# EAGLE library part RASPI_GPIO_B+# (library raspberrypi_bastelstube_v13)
2x20 header connector, all pins connected
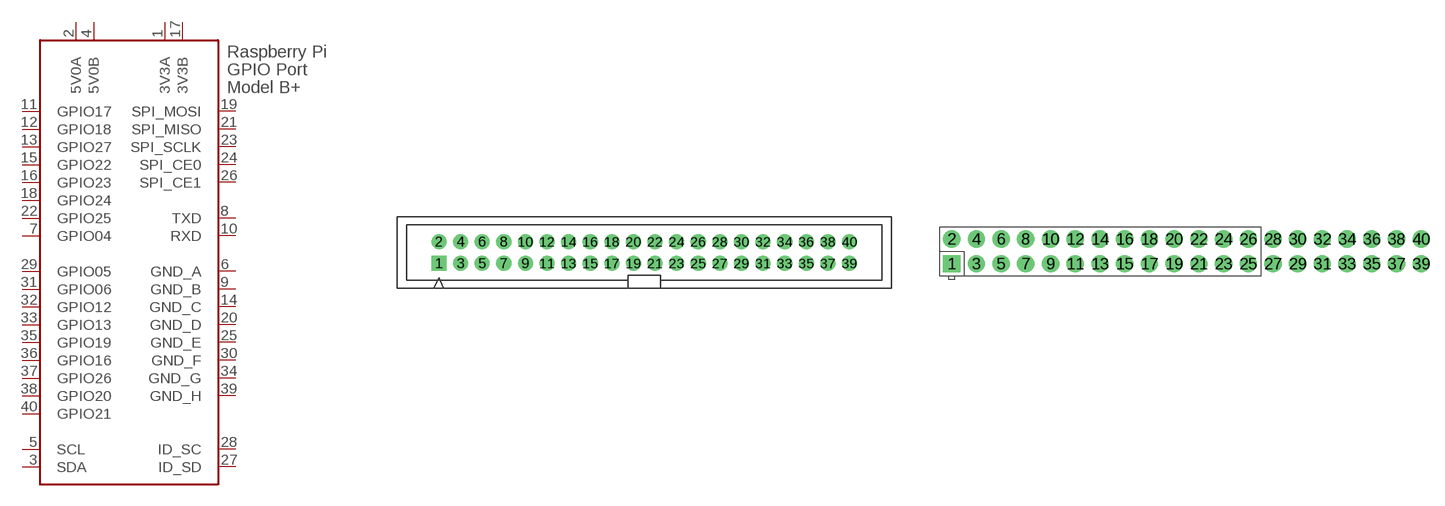
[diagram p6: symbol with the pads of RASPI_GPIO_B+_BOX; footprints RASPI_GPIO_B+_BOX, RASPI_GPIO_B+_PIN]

Designator prefix X

## RASPI_GPIO_B+#_BOX  [RASPI_GPIO_B+_BOX]
1  3V3A  pwr
2  5V0A  pwr
3  SDA
4  5V0B  pwr
5  SCL
6  GND_A  pwr
7  GPIO04
8  TXD
9  GND_B  pwr
10  RXD
11  GPIO17
12  GPIO18
13  GPIO27
14  GND_C  pwr
15  GPIO22
16  GPIO23
17  3V3B  pwr
18  GPIO24
19  SPI_MOSI
20  GND_D  pwr
21  SPI_MISO
22  GPIO25
23  SPI_SCLK
24  SPI_CE0
25  GND_E  pwr
26  SPI_CE1
27  ID_SD  nc
28  ID_SC  nc
29  GPIO05  nc
30  GND_F  pwr
31  GPIO06  nc
32  GPIO12  nc
33  GPIO13  nc
34  GND_G  pwr
35  GPIO19  nc
36  GPIO16  nc
37  GPIO26  nc
38  GPIO20  nc
39  GND_H  pwr
40  GPIO21  nc

## RASPI_GPIO_B+#_PIN  [RASPI_GPIO_B+_PIN]
Pads as for RASPI_GPIO_B+_BOX

## Footprint RASPI_GPIO_B+_BOX (pad centres in mm)
40-pin box header for Raspberry Pi GPIO model B+ for use with flat ribbon cables
drill 1 pad 1.778 square: 1 -24.13,-1.27
drill 1 pad 1.778: 2 -24.13,1.27; 3 -21.59,-1.27; 4 -21.59,1.27; 5 -19.05,-1.27; 6 -19.05,1.27; 7 -16.51,-1.27; 8 -16.51,1.27; 9 -13.97,-1.27; 10 -13.97,1.27; 11 -11.43,-1.27; 12 -11.43,1.27; 13 -8.89,-1.27; 14 -8.89,1.27; 15 -6.35,-1.27; 16 -6.35,1.27; 17 -3.81,-1.27; 18 -3.81,1.27; 19 -1.27,-1.27; 20 -1.27,1.27; 21 1.27,-1.27; 22 1.27,1.27; 23 3.81,-1.27; 24 3.81,1.27; 25 6.35,-1.27; 26 6.35,1.27; 27 8.89,-1.27; 28 8.89,1.27; 29 11.43,-1.27; 30 11.43,1.27; 31 13.97,-1.27; 32 13.97,1.27; 33 16.51,-1.27; 34 16.51,1.27; 35 19.05,-1.27; 36 19.05,1.27; 37 21.59,-1.27; 38 21.59,1.27; 39 24.13,-1.27; 40 24.13,1.27

## Footprint RASPI_GPIO_B+_PIN (pad centres in mm)
40-pin connector for Raspberry Pi GPIO model B+ just the two rows of pins
drill 1 pad 1.778 square: 1 -24.13,-1.27
drill 1 pad 1.778: 2 -24.13,1.27; 3 -21.59,-1.27; 4 -21.59,1.27; 5 -19.05,-1.27; 6 -19.05,1.27; 7 -16.51,-1.27; 8 -16.51,1.27; 9 -13.97,-1.27; 10 -13.97,1.27; 11 -11.43,-1.27; 12 -11.43,1.27; 13 -8.89,-1.27; 14 -8.89,1.27; 15 -6.35,-1.27; 16 -6.35,1.27; 17 -3.81,-1.27; 18 -3.81,1.27; 19 -1.27,-1.27; 20 -1.27,1.27; 21 1.27,-1.27; 22 1.27,1.27; 23 3.81,-1.27; 24 3.81,1.27; 25 6.35,-1.27; 26 6.35,1.27; 27 8.89,-1.27; 28 8.89,1.27; 29 11.43,-1.27; 30 11.43,1.27; 31 13.97,-1.27; 32 13.97,1.27; 33 16.51,-1.27; 34 16.51,1.27; 35 19.05,-1.27; 36 19.05,1.27; 37 21.59,-1.27; 38 21.59,1.27; 39 24.13,-1.27; 40 24.13,1.27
